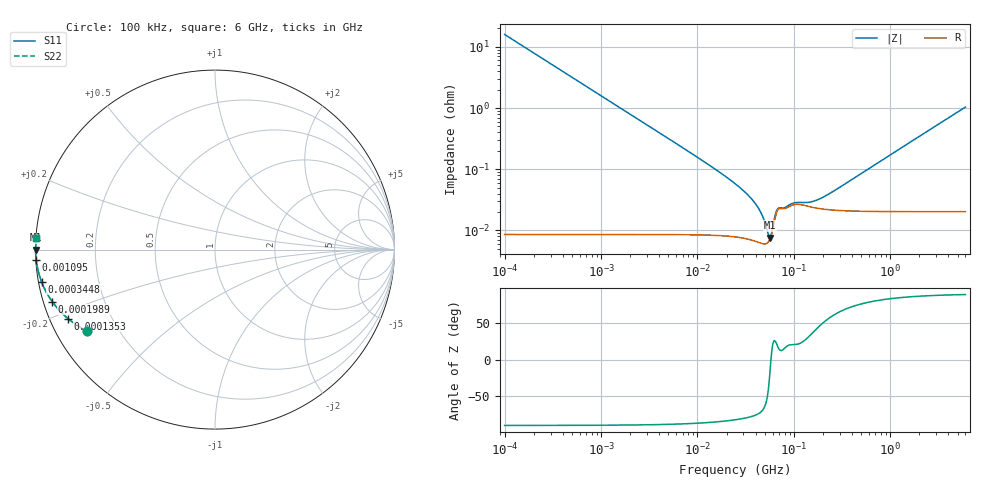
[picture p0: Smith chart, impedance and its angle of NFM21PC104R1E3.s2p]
! NFM21PC104R1E3
# Hz S RI R 50
!Freq.(Hz) S11(Real) S11(Imag) S21(Real) S21(Imag) S12(Real) S12(Imag) S22(Real) S22(Imag)
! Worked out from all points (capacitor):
!   401 points, 100 kHz to 6 GHz, reference 50 ohm
!   read as one part in shunt: C = 100 nF near 105.7 kHz
!   lowest |Z| = 7.66 mohm at 55.9 MHz (marker M1)
!   series resonance near 57.78 MHz, so ESL is about 76 pH
!   S11 on the Smith chart (normalised r, x): 100 kHz: 0.09, -0.29; 135.3 kHz: 0.05, -0.22; 198.9 kHz: 0.03, -0.16; 344.8 kHz: 0.01, -0.09; 1.095 MHz: 0.00, -0.03; 6 GHz: 0.00, +0.03
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100000  -0.7114 -0.4528  0.2885 -0.4528  0.2885 -0.4528  -0.7114 -0.4528
135331.6  -0.8185 -0.3849  0.1813 -0.3849  0.1813 -0.3849  -0.8185 -0.3849
198899.8  -0.9067 -0.2901  0.0932 -0.2901  0.0932 -0.2901  -0.9067 -0.2901
344780  -0.9666 -0.1784  0.0333 -0.1784  0.0333 -0.1784  -0.9666 -0.1784
631452  -0.9895 -0.0997  0.0104 -0.0997  0.0104 -0.0997  -0.9895 -0.0997
1094581  -0.9962 -0.0579  0.00371 -0.0579  0.00371 -0.0579  -0.9962 -0.0579
3987316  -0.9993 -0.0159  0.000595 -0.0159  0.000595 -0.0159  -0.9993 -0.0159
1.337449e7  -0.9995 -0.00454  0.000356 -0.00461  0.000356 -0.00461  -0.9995 -0.00454
2.517799e7  -0.9995 -0.0021  0.000317 -0.00223  0.000317 -0.00223  -0.9995 -0.0021
3.407377e7  -0.9996 -0.00127  0.000288 -0.00144  0.000288 -0.00144  -0.9996 -0.00127
4.130835e7  -0.9996 -0.000772  0.000262 -0.000979  0.000262 -0.000979  -0.9996 -0.000772
4.611257e7  -0.9996 -0.000475  0.000246 -0.000707  0.000246 -0.000707  -0.9996 -0.000475
5.291103e7  -0.9996 -4.76e-05  0.000249 -0.000314  0.000249 -0.000314  -0.9996 -4.76e-05
5.590324e7  -0.9996 0.000158  0.00028 -0.000124  0.00028 -0.000124  -0.9996 0.000158
5.906466e7  -0.9995 0.000382  0.000365 8.4e-05  0.000365 8.4e-05  -0.9995 0.000382
6.593397e7  -0.9991 0.000642  0.000773 0.000311  0.000773 0.000311  -0.9991 0.000642
6.966265e7  -0.9989 0.000588  0.0009 0.000238  0.0009 0.000238  -0.9989 0.000588
1.023848e8  -0.9987 0.000884  0.00106 0.000398  0.00106 0.000398  -0.9987 0.000884
1.546735e8  -0.9988 0.00136  0.000957 0.000693  0.000957 0.000693  -0.9988 0.00136
2.401829e8  -0.9989 0.0024  0.000869 0.00139  0.000869 0.00139  -0.9989 0.0024
9.76689e8  -0.9989 0.0108  0.000885 0.00666  0.000885 0.00666  -0.9989 0.0108
6e9  -0.9959 0.0666  0.00356 0.0412  0.00356 0.0412  -0.9959 0.0666
